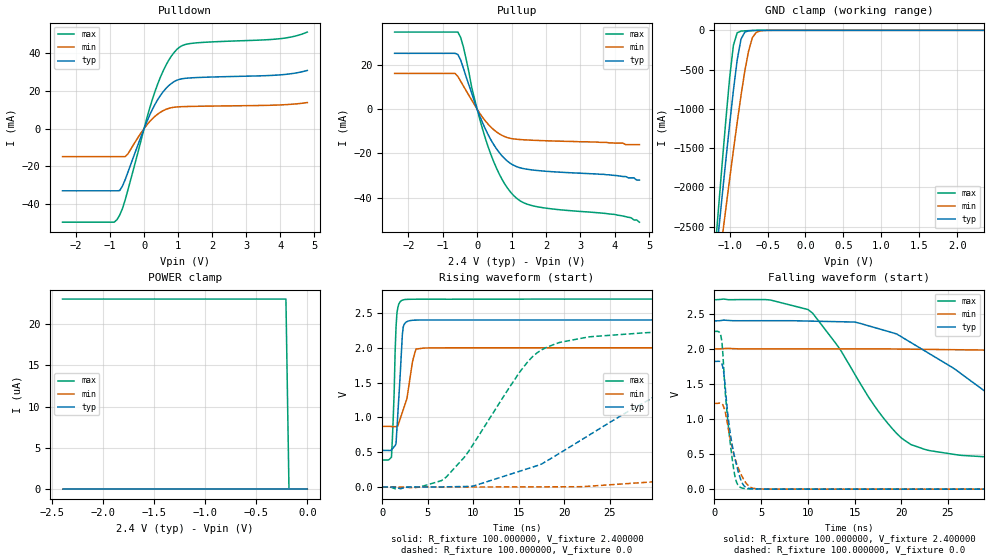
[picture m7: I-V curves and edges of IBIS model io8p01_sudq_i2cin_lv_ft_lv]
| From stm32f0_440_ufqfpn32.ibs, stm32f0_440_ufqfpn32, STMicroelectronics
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|   Model io8p01_sudq_i2cin_lv_ft_lv
[Model]  io8p01_sudq_i2cin_lv_ft_lv
Model_type I/O
Polarity   Non-Inverting
Enable   Active-Low
Vinl =   0.720000V
Vinh =   1.680000V
Vmeas =  1.200000V
Cref =   50.000000pF
Rref =   100.000000M
Vref =   0.0V
C_comp   2.067900pF   1.988600pF   2.164800pF
[Temperature Range]   25.000000   0.125000k   -40.000000
[Pullup Reference]   2.400000V   2.000000V   2.700000V
[Pulldown Reference]   0.0V   0.0V   0.0V
[POWER Clamp Reference]   2.400000V   2.000000V   2.700000V
[GND Clamp Reference]   0.0V   0.0V   0.0V
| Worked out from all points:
|   slope of the pulldown table from 0 to 0.36 V, typ, clamps not added: 25.5 ohm
|   slope of the pullup table from 0 to 0.36 V, typ, clamps not added: 28.4 ohm
|   GND clamp passes 1 mA (typ) near -0.64 V on its own axis
|   rising waveform, R_fixture 100.000000, V_fixture 2.400000: 20-80 % time 500ps typ, 1.02ns min, 334ps max; typ from 0.525 V to 2.4 V
|   rising waveform, R_fixture 100.000000, V_fixture 0.0: 20-80 % time 14.6ns typ, 43.1ns min, 6.86ns max; typ from 0 V to 1.82 V
|   falling waveform, R_fixture 100.000000, V_fixture 2.400000: 20-80 % time 12.8ns typ, 32.3ns min, 7.05ns max; typ from 2.4 V to 0.525 V
|   falling waveform, R_fixture 100.000000, V_fixture 0.0: 20-80 % time 1.17ns typ, 1.4ns min, 924ps max; typ from 1.82 V to 0 V
[Pulldown]
|Voltage   I(typ)   I(min)   I(max)
-2.4V     -33.16mA   -14.98mA   -49.86mA
-880mV    -33.16mA   -14.98mA   -49.86mA
-800mV    -33.16mA   -14.98mA   -48.55mA
-640mV    -30.75mA   -14.98mA   -42.76mA
-480mV    -23.43mA   -13.57mA   -32.92mA
80mV      3.651mA    1.905mA    5.506mA
400mV     15.37mA    7.665mA    23.73mA
720mV     22.75mA    10.69mA    36.23mA
1.04V     26.18mA    11.57mA    43.27mA
1.52V     27.09mA    11.81mA    45.55mA
4V        28.55mA    12.55mA    47.81mA
4.8V      30.9mA     13.81mA    51.31mA
[Pullup]
|Voltage   I(typ)   I(min)   I(max)
-2.4V     25.19mA    16.13mA    34.78mA
-640mV    25.19mA    16.13mA    34.78mA
-560mV    24.71mA    14.75mA    34.78mA
-400mV    18.52mA    10.48mA    28.1mA
-160mV    7.327mA    4.151mA    10.02mA
80mV      -3.229mA   -1.94mA    -4.736mA
400mV     -13.82mA   -8.08mA    -20.45mA
800mV     -22.31mA   -12.38mA   -33.66mA
1.2V      -26.24mA   -13.65mA   -40.82mA
1.76V     -27.69mA   -14.12mA   -44.06mA
4V        -29.9mA    -15.3mA    -47.5mA
4.72V     -32mA      -16mA      -51mA
[GND_clamp]
|Voltage   I(typ)   I(min)   I(max)
-2.4V     -9.567A    -9.921A    -9.731A
-1.2V     -3.09A     -3.428A    -2.911A
-1.15V    -2.606A    -3.04A     -2.31A
-1.1V     -2.127A    -2.655A    -1.719A
-1.05V    -1.657A    -2.274A    -1.146A
-950mV    -765.3mA   -1.53A     -190.2mA
-900mV    -376.6mA   -1.172A    -30.81mA
-850mV    -112.3mA   -832.5mA   -10.23mA
-750mV    -6.57mA    -264.6mA   -4.026mA
-700mV    -2.581mA   -94.26mA   -2.329mA
-600mV    -416.4uA   -8.158mA   -368uA
2.35V     0A         0A         0A
[POWER_clamp]
|Voltage   I(typ)   I(min)   I(max)
-2.4V     0A         0A         23.03uA
-210mV    0A         0A         23.03uA
-180mV    0A         0A         0A
0V        0A         0A         0A
[Ramp]
| variable   typ   min   max
dV/dt_r  1.09302/14.56747n   0.73368/43.04318n   1.34964/6.82906n
dV/dt_f  1.12490/12.82176n   0.67753/32.28059n   1.38749/7.04075n
R_load = 100.000000
[Rising Waveform]
R_fixture= 100.000000
V_fixture= 2.400000
V_fixture_min= 2.000000
V_fixture_max= 2.700000
|time   V(typ)   V(min)   V(max)
0s        525.2mV    870.3mV    387.4mV
1.001ns   533.3mV    868.7mV    427.5mV
1.301ns   579.6mV    867.1mV    1.371V
1.401ns   595mV      866.7mV    1.927V
1.502ns   617.8mV    866.4mV    2.293V
1.702ns   1.049V     877mV      2.578V
2.202ns   2.195V     1.073V     2.684V
2.603ns   2.367V     1.23V      2.695V
3.704ns   2.398V     1.982V     2.698V
49.85ns   2.4V       2V         2.7V
[Rising Waveform]
R_fixture= 100.000000
V_fixture= 0.0
V_fixture_min= 0.0
V_fixture_max= 0.0
|time   V(typ)   V(min)   V(max)
0s        1.475nV    15.65nV    1.121nV
7.007ns   1.813mV    -87.46uV   139.2mV
15.02ns   222mV      830.7uV    1.635V
17.52ns   329.4mV    1.729mV    1.97V
29.03ns   1.23V      66.77mV    2.217V
35.54ns   1.585V     124.9mV    2.234V
45.05ns   1.742V     261.9mV    2.247V
88.59ns   1.821V     999.2mV    2.249V
102.6ns   1.822V     1.113V     2.249V
249.2ns   1.822V     1.223V     2.249V
[Falling Waveform]
R_fixture= 100.000000
V_fixture= 2.400000
V_fixture_min= 2.000000
V_fixture_max= 2.700000
|time   V(typ)   V(min)   V(max)
0s        2.4V       2V         2.7V
10.01ns   2.397V     2V         2.561V
15.02ns   2.383V     2V         1.64V
20.02ns   2.171V     1.997V     729mV
26.53ns   1.634V     1.987V     480.9mV
36.04ns   829.7mV    1.955V     421.3mV
51.05ns   601mV      1.703V     395.5mV
76.58ns   543.7mV    1.143V     387.7mV
100.1ns   527.8mV    964.4mV    387.5mV
249.2ns   525.2mV    870.3mV    387.4mV
[Falling Waveform]
R_fixture= 100.000000
V_fixture= 0.0
V_fixture_min= 0.0
V_fixture_max= 0.0
|time   V(typ)   V(min)   V(max)
0s        1.822V     1.223V     2.249V
700.7ps   1.802V     1.223V     2.18V
1.001ns   1.656V     1.166V     1.711V
1.401ns   1.099V     926.8mV    1.011V
1.902ns   625.9mV    597.7mV    432.4mV
2.302ns   377.6mV    393.7mV    125.3mV
2.903ns   106.7mV    196.5mV    18.39mV
3.704ns   11.55mV    40.86mV    3.593mV
5.105ns   1.697mV    2.513mV    1.193mV
49.85ns   1.475nV    15.65nV    1.121nV
